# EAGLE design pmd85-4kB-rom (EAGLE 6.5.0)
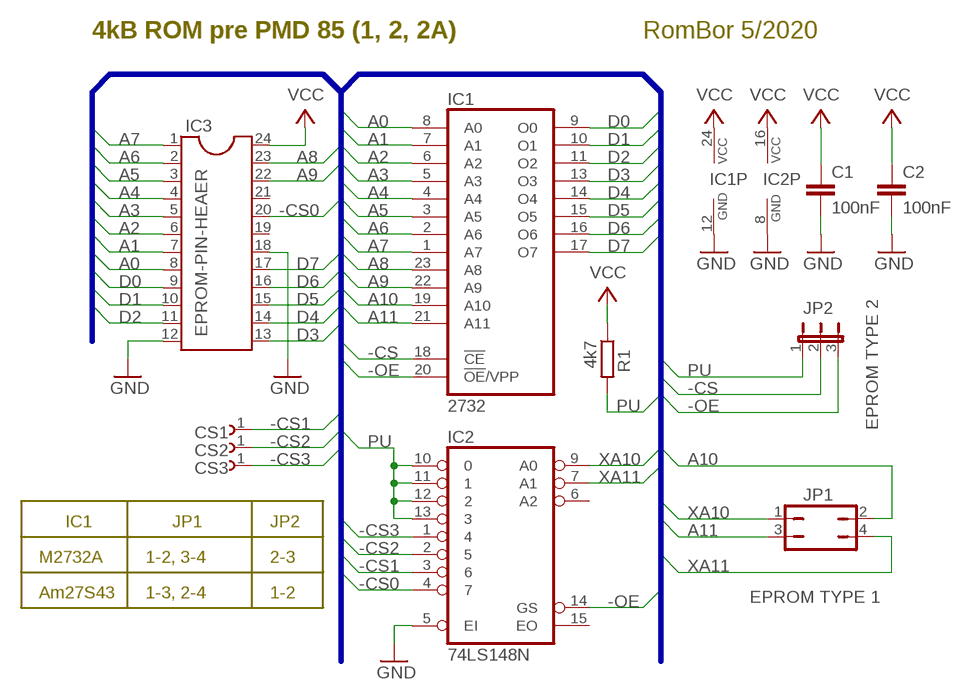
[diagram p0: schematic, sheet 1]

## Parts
C1  100nF  C2.5/2  [C2.5-2]
C2  100nF  C2.5/2  [C2.5-2]
CS1  CS1  PINHD-1X1  [1X01]
CS2  CS2  PINHD-1X1  [1X01]
CS3  CS3  PINHD-1X1  [1X01]
IC1  2732  [DIL24]
IC2  74LS148N  [DIL16]
IC3  EPROM-PIN-HEAER  DIL24-6  [DIL24-6]
JP1  EPROM TYPE 1  JP2Q  [JP2Q]
JP2  EPROM TYPE 2  JP2E  [JP2]
R1  4k7  R-EU_0207/10  [0207/10]

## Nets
-CS: IC1.18(!CE) JP2.2
-CS0: IC2.4 IC3.20
-CS1: CS1.1 IC2.3
-CS2: CS2.1 IC2.2
-CS3: CS3.1 IC2.1
-OE: IC1.20(!OE!/VPP) IC2.14(GS) JP2.3
A0: IC1.8(A0) IC3.8
A1: IC1.7(A1) IC3.7
A2: IC1.6(A2) IC3.6
A3: IC1.5(A3) IC3.5
A4: IC1.4(A4) IC3.4
A5: IC1.3(A5) IC3.3
A6: IC1.2(A6) IC3.2
A7: IC1.1(A7) IC3.1
A8: IC1.23(A8) IC3.23
A9: IC1.22(A9) IC3.22
A10: IC1.19(A10) JP1.2
A11: IC1.21(A11) JP1.3
D0: IC1.9(O0) IC3.9
D1: IC1.10(O1) IC3.10
D2: IC1.11(O2) IC3.11
D3: IC1.13(O3) IC3.13
D4: IC1.14(O4) IC3.14
D5: IC1.15(O5) IC3.15
D6: IC1.16(O6) IC3.16
D7: IC1.17(O7) IC3.17
GND: C1.2 C2.2 IC1.12(GND) IC2.5(EI) IC2.8(GND) IC3.12 IC3.18
PU: IC2.10 IC2.11 IC2.12 IC2.13 JP2.1 R1.2
VCC: C1.1 C2.1 IC1.24(VCC) IC2.16(VCC) IC3.24 R1.1
XA10: IC2.9(A0) JP1.1
XA11: IC2.7(A1) JP1.4
Unconnected: IC2.6(A2) IC2.15(EO) IC3.19 IC3.21

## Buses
A[0..11],D[0..7],-CS[0..3],-CS,-OE,XA10,XA11,PU

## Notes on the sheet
- 4kB ROM pre PMD 85 (1, 2, 2A) | RomBor 5/2020
- IC1 | JP1 | JP2
- M2732A | 1-2, 3-4 | 2-3
- Am27S43 | 1-3, 2-4 | 1-2

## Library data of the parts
C1 C2 = capacitor-wima:C: CAPACITOR
CS1-CS3 = pinhead_MP_08mm:PINHD-1X1: PIN HEADER
IC1 = memory:2732: MEMORY
IC2 = 74xx-eu:74*148: 10-line to 4-line and 8-line to 3-line PRIORITY ENCODER
IC3 = ic-package:DIL24: Dual In Line
JP1 = jumper:JP2Q: JUMPER
JP2 = jumper:JP2E: JUMPER
R1 = rcl:R-EU_: RESISTOR, European symbol

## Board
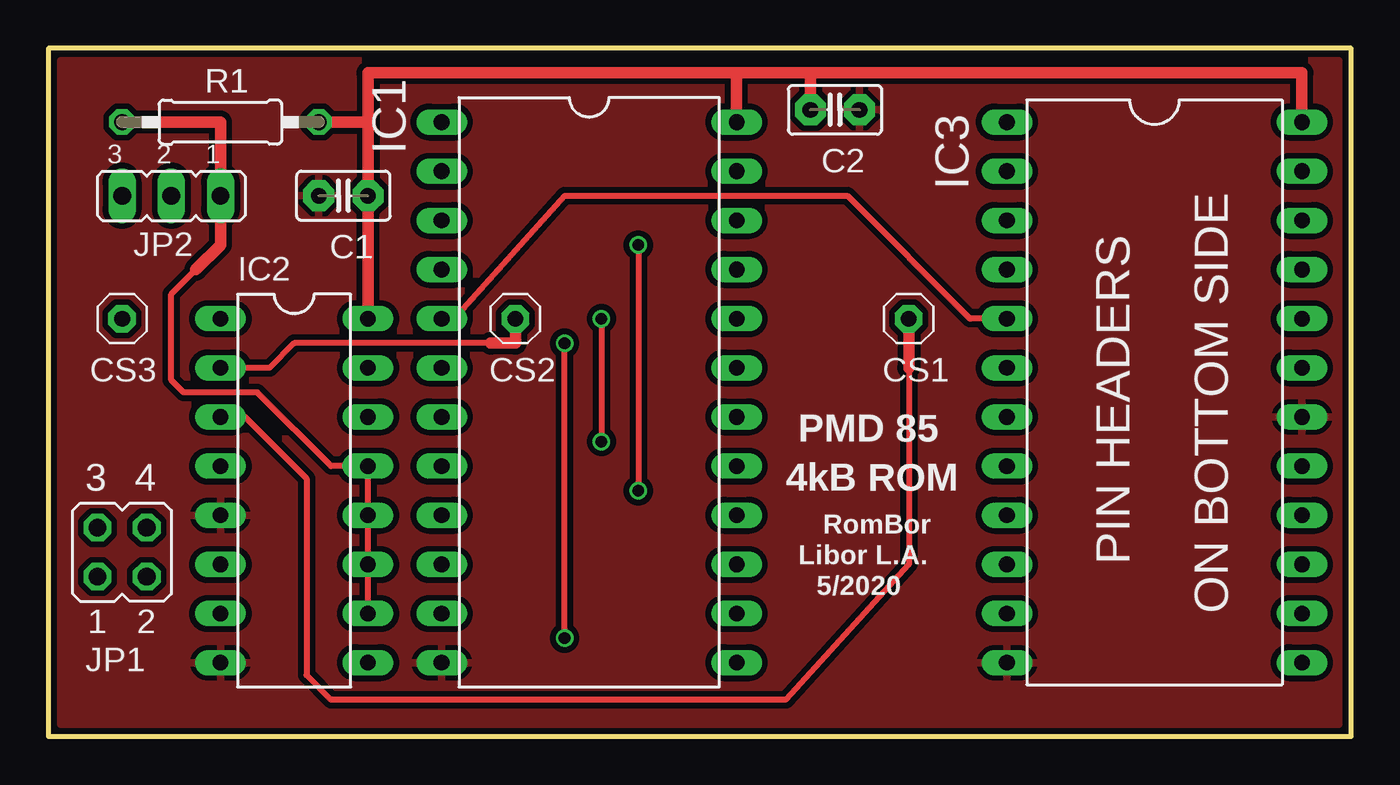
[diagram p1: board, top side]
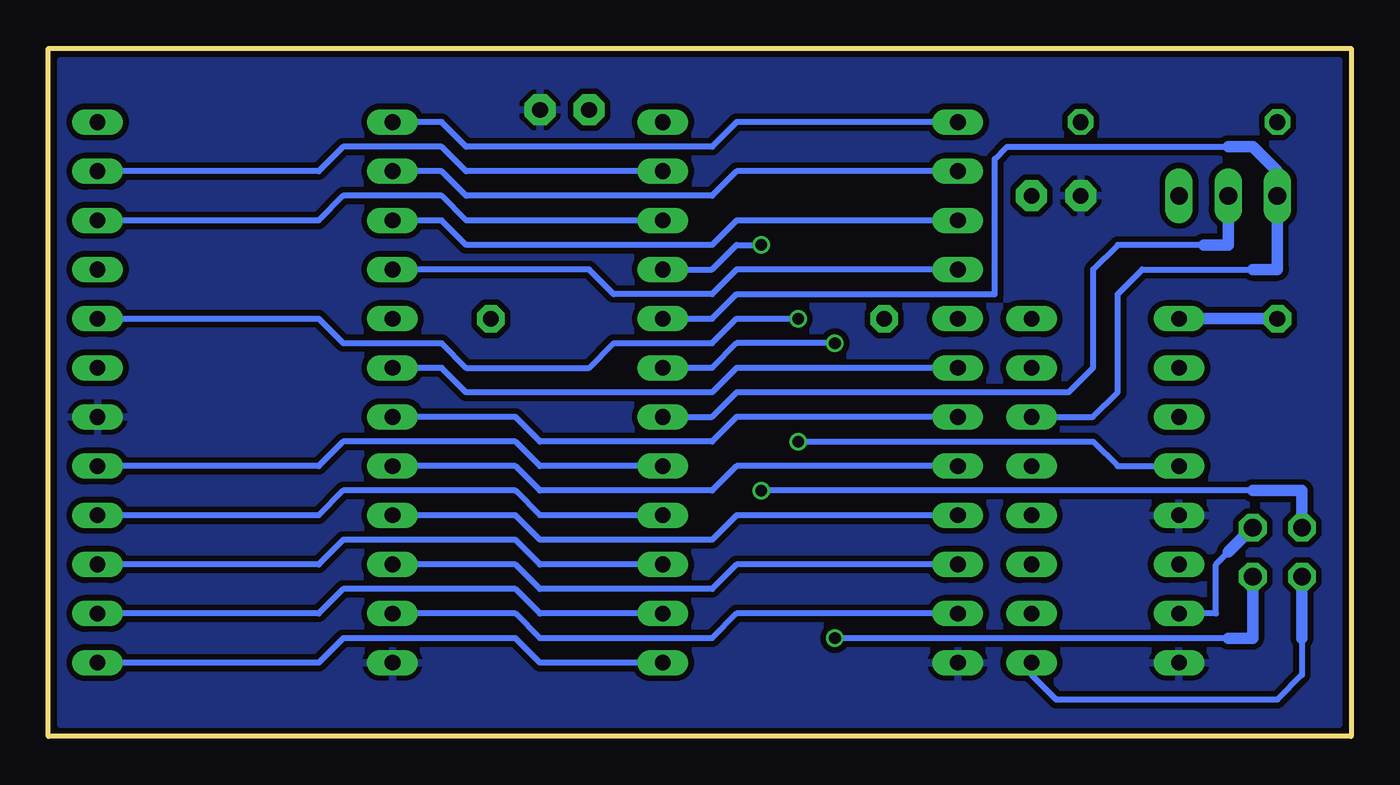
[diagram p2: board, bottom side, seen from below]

Size 67.31 x 35.56 mm. Coordinates in mm from the lower left corner, seen from the top.
Outline: 0,0 67.31,0 67.31,35.56 0,35.56 0,0
Copper layers (1*16): Top 0.035mm / dielectric 1.5mm / Bottom 0.035mm
Design rules "SeeedStudio_2layer_DRU_no_angle_20140221": minimum track width 6mil, minimum drill 12mil, track to track 6mil, track to pad 6mil, pad to pad 6mil, via to via 6mil, smd to smd 0mil, copper to edge 10mil, drill to drill 10mil, minimum pad ring 10mil, minimum via ring 6mil, stop-mask expansion 2mil, vias tented up to drill 100mil, thermal gap 10mil

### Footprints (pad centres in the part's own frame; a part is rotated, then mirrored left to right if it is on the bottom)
C2.5-2 = drill 0.813 pad 1.6 octagon: 1 -1.27,0; 2 1.27,0
1X01 = drill 0.813 pad 1.422 octagon: 1 0,0
DIL24 = drill 0.813 long: 1 -13.97,-7.62; 2 -11.43,-7.62; 3 -8.89,-7.62; 4 -6.35,-7.62; 5 -3.81,-7.62; 6 -1.27,-7.62; 7 1.27,-7.62; 8 3.81,-7.62; 9 6.35,-7.62; 10 8.89,-7.62; 11 11.43,-7.62; 12 13.97,-7.62; 13 13.97,7.62; 14 11.43,7.62; 15 8.89,7.62; 16 6.35,7.62; 17 3.81,7.62; 18 1.27,7.62; 19 -1.27,7.62; 20 -3.81,7.62; 21 -6.35,7.62; 22 -8.89,7.62; 23 -11.43,7.62; 24 -13.97,7.62
DIL16 = drill 0.813 long: 1 -8.89,-3.81; 2 -6.35,-3.81; 3 -3.81,-3.81; 4 -1.27,-3.81; 5 1.27,-3.81; 6 3.81,-3.81; 7 6.35,-3.81; 8 8.89,-3.81; 9 8.89,3.81; 10 6.35,3.81; 11 3.81,3.81; 12 1.27,3.81; 13 -1.27,3.81; 14 -3.81,3.81; 15 -6.35,3.81; 16 -8.89,3.81
DIL24-6 = drill 0.813 long: 1 -13.97,-7.62; 2 -11.43,-7.62; 3 -8.89,-7.62; 4 -6.35,-7.62; 5 -3.81,-7.62; 6 -1.27,-7.62; 7 1.27,-7.62; 8 3.81,-7.62; 9 6.35,-7.62; 10 8.89,-7.62; 11 11.43,-7.62; 12 13.97,-7.62; 13 13.97,7.62; 14 11.43,7.62; 15 8.89,7.62; 16 6.35,7.62; 17 3.81,7.62; 18 1.27,7.62; 19 -1.27,7.62; 20 -3.81,7.62; 21 -6.35,7.62; 22 -8.89,7.62; 23 -11.43,7.62; 24 -13.97,7.62
JP2Q = drill 0.914 octagon: 1 -1.27,-1.27; 2 1.27,-1.27; 3 -1.27,1.27; 4 1.27,1.27
JP2 = drill 0.914 long: 1 -2.54,0; 2 0,0; 3 2.54,0
0207/10 = drill 0.813 octagon: 1 -5.08,0; 2 5.08,0

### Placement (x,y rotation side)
C1  15.24,27.94 180 top
C2  40.64,32.38 0 top
CS1  44.45,21.59 0 top
CS2  24.13,21.59 0 top
CS3  3.81,21.59 0 top
IC1  27.94,17.78 270 top
IC2  12.7,12.7 270 top
IC3  57.15,17.78 270 top
JP1  3.81,9.53 0 top
JP2  6.35,27.94 180 top
R1  8.89,31.75 180 top

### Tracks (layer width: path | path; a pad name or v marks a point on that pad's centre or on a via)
-CS
  Bottom 0.3: IC1.18 33.02,16.51 31.75,17.78 14.61,17.78 13.34,19.05 13.34,24.13 12.06,25.4 7.62,25.4
  Bottom 0.6: JP2.2 6.35,25.4 7.62,25.4
-CS0  (via drill 0.6)
  Top 0.3: v28.57,21.59 v28.57,15.24
  Bottom 0.3: IC3.20 53.34,21.59 52.07,20.32 46.99,20.32 45.72,19.05 39.37,19.05 38.1,20.32 33.02,20.32 31.75,21.59 v28.57,21.59 | v28.57,15.24 13.34,15.24 12.06,13.97 IC2.4
-CS1
  Top 0.3: 44.45,19.05 44.45,8.89 38.1,1.91 14.61,1.91 13.34,3.17 13.34,13.34 10.16,16.51 IC2.3
  Top 0.6: CS1.1 44.45,19.05
-CS2
  Top 0.3: 22.86,20.32 12.7,20.32 11.43,19.05 IC2.2
  Top 0.6: CS2.1 24.13,20.32 22.86,20.32
-CS3
  Bottom 0.6: CS3.1 IC2.1
-OE
  Bottom 0.3: IC2.14 13.34,16.51 12.06,17.78 12.06,22.86 10.79,24.13 5.08,24.13 | IC1.20 33.02,21.59 31.75,22.86 18.41,22.86 18.41,29.84 17.78,30.48 6.35,30.48
  Bottom 0.6: 5.08,24.13 3.81,24.13 JP2.3 3.81,29.21 5.08,30.48 6.35,30.48
A0
  Bottom 0.3: IC1.8 31.75,13.97 33.02,12.7 41.91,12.7 43.18,13.97 IC3.8
A1
  Bottom 0.3: IC1.7 31.75,16.51 33.02,15.24 41.91,15.24 43.18,16.51 IC3.7
A2
  Bottom 0.3: IC1.6 31.75,19.05 33.02,17.78 45.72,17.78 46.99,19.05 IC3.6
A3
  Top 0.3: IC1.5 20.95,21.59 26.67,27.94 41.27,27.94 47.62,21.59 IC3.5
A4
  Bottom 0.3: IC1.4 31.75,24.13 33.02,22.86 38.1,22.86 39.37,24.13 IC3.4
A5
  Bottom 0.3: IC1.3 31.75,26.67 33.02,25.4 45.72,25.4 46.99,26.67 IC3.3
A6
  Bottom 0.3: IC1.2 31.75,29.21 33.02,27.94 45.72,27.94 46.99,29.21 IC3.2
A7
  Bottom 0.3: IC1.1 31.75,31.75 33.02,30.48 45.72,30.48 46.99,31.75 IC3.1
A8
  Bottom 0.3: IC1.23 45.72,29.21 46.99,30.48 52.07,30.48 53.34,29.21 IC3.23
A9
  Bottom 0.3: IC1.22 45.72,26.67 46.99,27.94 52.07,27.94 53.34,26.67 IC3.22
A10  (via drill 0.6)
  Top 0.3: v26.67,5.08 v26.67,20.32
  Bottom 0.3: 6.35,5.08 v26.67,5.08 | v26.67,20.32 31.75,20.32 33.02,19.05 IC1.19
  Bottom 0.6: JP1.2 5.08,5.08 6.35,5.08
A11  (via drill 0.6)
  Top 0.3: v30.48,25.4 v30.48,12.7
  Bottom 0.3: IC1.21 33.02,24.13 31.75,25.4 v30.48,25.4 | 5.08,12.7 v30.48,12.7
  Bottom 0.6: 5.08,12.7 2.54,12.7 JP1.3
D0
  Bottom 0.3: IC1.9 31.75,11.43 33.02,10.16 41.91,10.16 43.18,11.43 IC3.9
D1
  Bottom 0.3: IC1.10 31.75,8.89 33.02,7.62 41.91,7.62 43.18,8.89 IC3.10
D2
  Bottom 0.3: IC1.11 31.75,6.35 33.02,5.08 41.91,5.08 43.18,6.35 IC3.11
D3
  Bottom 0.3: IC1.13 41.91,3.81 43.18,5.08 52.07,5.08 53.34,3.81 IC3.13
D4
  Bottom 0.3: IC1.14 41.91,6.35 43.18,7.62 52.07,7.62 53.34,6.35 IC3.14
D5
  Bottom 0.3: IC1.15 41.91,8.89 43.18,10.16 52.07,10.16 53.34,8.89 IC3.15
D6
  Bottom 0.3: IC1.16 41.91,11.43 43.18,12.7 52.07,12.7 53.34,11.43 IC3.16
D7
  Bottom 0.3: IC1.17 41.91,13.97 43.18,15.24 52.07,15.24 53.34,13.97 IC3.17
GND
  pour Top (isolate 0.3): 0.64,34.92 66.67,34.92 66.67,0.64 0.64,0.64
  pour Bottom (isolate 0.3): 0.64,34.92 0.64,0.64 66.67,0.64 66.67,34.92
PU
  Top 0.3: IC2.10 IC2.11 IC2.12 IC2.13 14.61,13.97 10.79,17.78 6.99,17.78 6.35,18.41 6.35,22.86 7.62,24.13
  Top 0.6: 7.62,24.13 8.89,25.4 JP2.1 8.89,31.75 R1.2
VCC
  Top 0.6: IC2.16 C1.1 16.51,31.75 | IC3.24 64.77,34.29 39.37,34.29 | 39.37,34.29 35.56,34.29 | 35.56,34.29 16.51,34.29 16.51,31.75 | 39.37,34.29 C2.1 | R1.1 16.51,31.75 | IC1.24 35.56,34.29
XA10
  Bottom 0.3: 2.54,5.08 2.54,3.17 3.81,1.91 15.24,1.91 16.51,3.17 IC2.9
  Bottom 0.6: JP1.1 2.54,5.08
XA11
  Bottom 0.3: IC2.7 6.99,6.35 6.99,8.89 6.35,9.53
  Bottom 0.6: 6.35,9.53 JP1.4

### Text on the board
tPlace: PMD 85 | 3 | 4 | 4kB ROM | RomBor | Libor L.A. | PIN HEADERS | 5/2020 | ON BOTTOM SIDE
